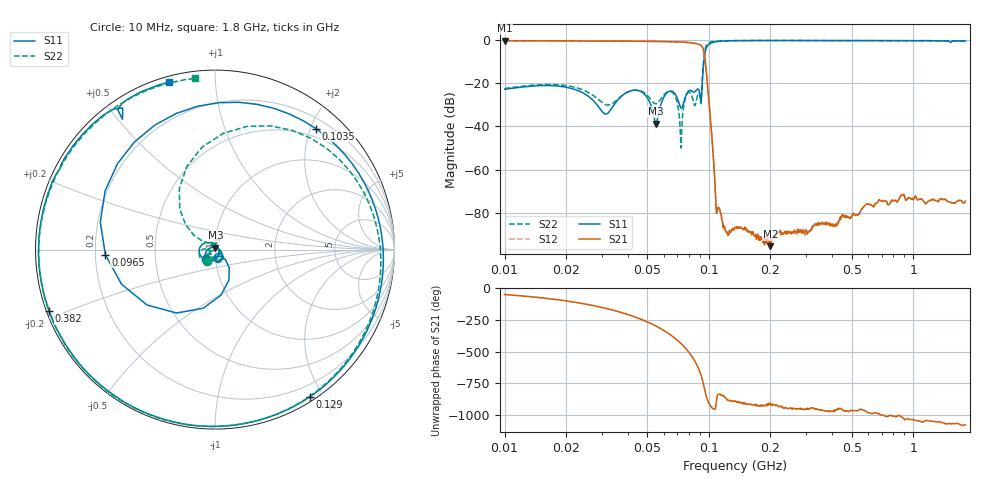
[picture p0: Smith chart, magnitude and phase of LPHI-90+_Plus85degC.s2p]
! Mini-Circuits
! S2P DATA File Format
! Type:LOW PASS FILTER
! Model: LPHI-90+
! All S Parameters are in dB deg format
! TEST CONDITIONS: INPUT POWER = 0 dBm,  +85deg C
# MHz S DB R 50
!Frequency  S11 dB  S11 DEG  S21 dB  S21 DEG  S12 dB  S12 DEG  S22 dB  S22 DEG
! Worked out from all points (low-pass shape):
!   493 points, 10 MHz to 1.8 GHz, reference 50 ohm
!   highest |S21| = -0.20 dB at 10 MHz (marker M1); lowest = -95.5 dB at 200 MHz (marker M2)
!   |S21| within 3 dB of the highest: start of sweep to 92.99 MHz
!   lowest |S11| = -38.6 dB at 55 MHz (marker M3), VSWR 1.02, Z = 50.2 + j1.16 ohm
!   |S11| at or under -10 dB: start of sweep to 94.4 MHz
!   |S22| runs from -50.0 to -0.1 dB; largest |S21 - S12| = 0.0009
!   S11 on the Smith chart (normalised r, x): 10 MHz: 0.90, -0.10; 96.5 MHz: 0.24, -0.02; 103.5 MHz: 0.36, +2.08; 129 MHz: 0.05, -1.83; 382 MHz: 0.01, -0.18; 1.8 GHz: 0.03, +0.76
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10  -22.73 -133.1  -0.20 -50.1  -0.19 -50.1  -22.40 -124.1
24  -24.24 138.6  -0.29 -120.6  -0.29 -120.6  -22.90 -179.9
38  -25.33 -84.0  -0.37 164.4  -0.37 164.5  -25.31 -123.8
47  -24.06 -149.8  -0.45 112.4  -0.45 112.4  -23.74 -145.4
55  -38.63 80.5  -0.52 62.1  -0.52 62.1  -29.47 -124.4
56.5  -34.67 17.0  -0.54 52.1  -0.53 52.1  -28.79 -110.9
67  -24.02 -83.1  -0.70 -24.5  -0.70 -24.4  -24.71 -130.8
73  -31.49 -70.6  -0.83 -75.7  -0.82 -75.6  -50.03 -80.8
82  -23.40 -57.4  -1.19 -170.2  -1.18 -170.2  -25.12 -93.2
88  -22.59 -69.4  -1.70 103.9  -1.70 104.0  -25.39 85.8
92.5  -21.65 -44.1  -2.85 9.4  -2.85 9.4  -20.90 146.3
96.5  -4.27 -177.3  -11.85 -115.9  -11.85 -115.9  -2.98 75.4
99.5  -2.06 105.9  -25.80 -178.3  -25.82 -178.3  -1.22 30.4
103.5  -1.13 50.2  -45.49 138.7  -45.50 138.8  -0.68 -2.6
109  -0.64 8.0  -80.20 -158.8  -80.39 -159.2  -0.41 -29.9
129  -0.21 -57.2  -88.17 -168.6  -87.86 -161.3  -0.16 -77.4
135  -0.18 -67.6  -87.03 -166.2  -86.67 -168.7  -0.14 -85.7
200  -0.10 -120.1  -95.54 173.4  -92.36 159.9  -0.08 -128.6
320  -0.12 -150.9  -86.55 137.6  -86.92 140.0  -0.12 -155.7
382  -0.13 -159.8  -84.70 113.2  -85.04 112.6  -0.12 -163.9
760  -0.16 169.6  -76.36 75.9  -76.40 76.8  -0.20 166.6
1800  -0.28 105.3  -74.65 3.2  -74.72 4.1  -0.35 96.5
